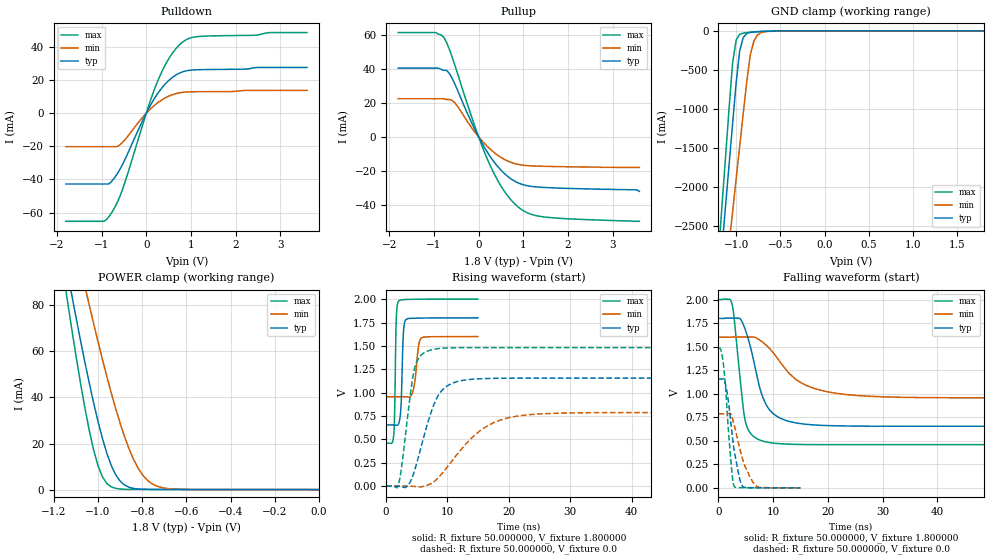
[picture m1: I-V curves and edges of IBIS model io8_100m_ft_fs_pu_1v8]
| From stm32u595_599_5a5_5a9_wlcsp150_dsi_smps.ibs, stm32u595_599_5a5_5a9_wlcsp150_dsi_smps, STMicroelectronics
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|   Model io8_100m_ft_fs_pu_1v8
[Model]  io8_100m_ft_fs_pu_1v8
Model_type I/O
Polarity   Non-Inverting
Enable   Active-Low
Vinl =   0.540000V
Vinh =   1.260000V
Vmeas =  0.900000V
Cref =   50.000000pF
Rref =   100.000000M
Vref =   0.0V
C_comp   3.148300pF   3.147400pF   3.196500pF
[Temperature Range]   25.000000   0.140000k   -40.000000
[Pullup Reference]   1.800000V   1.600000V   2.000000V
[Pulldown Reference]   0.0V   0.0V   0.0V
[POWER Clamp Reference]   1.800000V   1.600000V   2.000000V
[GND Clamp Reference]   0.0V   0.0V   0.0V
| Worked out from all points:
|   slope of the pulldown table from 0 to 0.27 V, typ, clamps not added: 21.7 ohm
|   slope of the pullup table from 0 to 0.27 V, typ, clamps not added: 22.6 ohm
|   GND clamp passes 1 mA (typ) near -0.51 V on its own axis
|   POWER clamp passes 1 mA (typ) near -0.86 V on its own axis
|   rising waveform, R_fixture 50.000000, V_fixture 1.800000: 20-80 % time 320ps typ, 635ps min, 232ps max; typ from 0.655 V to 1.8 V
|   rising waveform, R_fixture 50.000000, V_fixture 0.0: 20-80 % time 3.21ns typ, 6.76ns min, 1.69ns max; typ from 0.001 V to 1.16 V
|   falling waveform, R_fixture 50.000000, V_fixture 1.800000: 20-80 % time 3.22ns typ, 6.73ns min, 1.66ns max; typ from 1.8 V to 0.655 V
|   falling waveform, R_fixture 50.000000, V_fixture 0.0: 20-80 % time 1.6ns typ, 2.38ns min, 1.14ns max; typ from 1.16 V to 0.001 V
[Pulldown]
|Voltage   I(typ)   I(min)   I(max)
-1.8V     -42.74mA   -20.21mA   -65.25mA
-960mV    -42.74mA   -20.21mA   -65.25mA
-780mV    -41.3mA    -20.21mA   -60.25mA
-660mV    -37mA      -20.2mA    -54.5mA
-540mV    -31.39mA   -17.82mA   -46.65mA
0V        0A         0A         0A
240mV     11.28mA    6.002mA    18.38mA
480mV     19.17mA    10.02mA    31.83mA
780mV     24.67mA    12.5mA     42.21mA
960mV     25.9mA     12.9mA     45.21mA
1.2V      26.29mA    13.01mA    46.37mA
3.6V      27.65mA    13.81mA    48.71mA
[Pullup]
|Voltage   I(typ)   I(min)   I(max)
-1.8V     40.31mA    22.36mA    61.21mA
-960mV    40.31mA    22.36mA    61.21mA
-780mV    39.02mA    22.36mA    58.45mA
-660mV    37.4mA     21.91mA    51.75mA
-540mV    31.51mA    20.18mA    42.77mA
-120mV    6.338mA    4.065mA    8.965mA
240mV     -10.82mA   -6.752mA   -15.73mA
540mV     -20.62mA   -12.68mA   -30.5mA
900mV     -27.22mA   -16.28mA   -41.49mA
1.14V     -28.94mA   -17mA      -45.14mA
1.5V      -29.77mA   -17.34mA   -47.14mA
3.6V      -32mA      -18mA      -49.6mA
[GND_clamp]
|Voltage   I(typ)   I(min)   I(max)
-1.8V     -9.707A    -9.942A    -9.774A
-1.2V     -3.309A    -4.006A    -2.864A
-1.16V    -2.777A    -3.584A    -2.239A
-1.12V    -2.246A    -3.162A    -1.614A
-1.04V    -1.186A    -2.319A    -408.6mA
-1V       -663.9mA   -1.898A    -117.8mA
-960mV    -254mA     -1.478A    -45.14mA
-920mV    -86.03mA   -1.06A     -28.58mA
-840mV    -19.12mA   -308.9mA   -18.74mA
-800mV    -13.39mA   -130.8mA   -15.31mA
-720mV    -7.948mA   -25.37mA   -9.381mA
1.8V      0A         14.97nA    0A
[POWER_clamp]
|Voltage   I(typ)   I(min)   I(max)
-1.8V     470.9mA    433.7mA    554.6mA
-1.14V    95.28mA    122.7mA    82.88mA
-1.12V    85mA       114mA      70.34mA
-1.06V    55.55mA    88.43mA    35.73mA
-1.04V    46.38mA    80.17mA    25.83mA
-1V       29.54mA    64.14mA    10.37mA
-940mV    10.43mA    41.88mA    1.177mA
-900mV    3.66mA     28.79mA    250.5uA
-840mV    527.2uA    13.26mA    95.74uA
-800mV    153.8uA    6.55mA     88.56uA
-740mV    60.02uA    1.742mA    70.74uA
0V        0A         18.15nA    0A
[Ramp]
| variable   typ   min   max
dV/dt_r  0.69287/3.20311n   0.47204/6.75401n   0.88855/1.69005n
dV/dt_f  0.68715/3.21718n   0.38638/6.72632n   0.92438/1.65066n
R_load = 50.000000
[Rising Waveform]
R_fixture= 50.000000
V_fixture= 1.800000
V_fixture_min= 1.600000
V_fixture_max= 2.000000
|time   V(typ)   V(min)   V(max)
0s        654.8mV    956mV      459.4mV
1.231ns   654.6mV    956mV      544.2mV
1.652ns   651.7mV    956mV      1.793V
2.012ns   664.5mV    956.1mV    1.977V
2.402ns   832.9mV    956.1mV    1.991V
2.823ns   1.647V     955.9mV    1.995V
3.213ns   1.78V      954.9mV    1.996V
4.414ns   1.795V     1.027V     1.998V
5.646ns   1.798V     1.579V     1.999V
14.95ns   1.8V       1.6V       2V
[Rising Waveform]
R_fixture= 50.000000
V_fixture= 0.0
V_fixture_min= 0.0
V_fixture_max= 0.0
|time   V(typ)   V(min)   V(max)
0s        614.9uV    691.2uV    580.4uV
2.002ns   -968.9uV   688.6uV    15.4mV
3.804ns   30.98mV    55.73uV    908mV
5.005ns   250.6mV    -5.37mV    1.332V
7.608ns   841.7mV    37.87mV    1.462V
9.009ns   1.018V     127.3mV    1.474V
11.41ns   1.115V     327mV      1.48V
16.22ns   1.151V     632.5mV    1.481V
22.22ns   1.155V     756.5mV    1.481V
99.7ns    1.155V     787.4mV    1.481V
[Falling Waveform]
R_fixture= 50.000000
V_fixture= 1.800000
V_fixture_min= 1.600000
V_fixture_max= 2.000000
|time   V(typ)   V(min)   V(max)
0s        1.8V       1.6V       2V
2.202ns   1.804V     1.6V       1.998V
2.603ns   1.804V     1.602V     1.917V
4.404ns   1.753V     1.603V     906.3mV
5.005ns   1.662V     1.602V     684.2mV
8.408ns   920.2mV    1.531V     491.8mV
10.61ns   762.9mV    1.39V      472mV
14.81ns   684.2mV    1.127V     461.7mV
23.62ns   657.4mV    989.7mV    459.4mV
99.7ns    654.8mV    956mV      459.4mV
[Falling Waveform]
R_fixture= 50.000000
V_fixture= 0.0
V_fixture_min= 0.0
V_fixture_max= 0.0
|time   V(typ)   V(min)   V(max)
0s        1.155V     787.4mV    1.481V
420.4ps   1.155V     787.4mV    1.468V
930.9ps   1.16V      787.4mV    1.299V
1.562ns   1.016V     787.3mV    826.7mV
2.342ns   646.4mV    770.7mV    236.8mV
2.613ns   509.5mV    723.7mV    81.98mV
2.853ns   406.1mV    672.1mV    19.92mV
4.234ns   31.46mV    340.7mV    2.097mV
6.757ns   1.886mV    25.87mV    1.027mV
14.95ns   614.9uV    691.2uV    580.4uV
